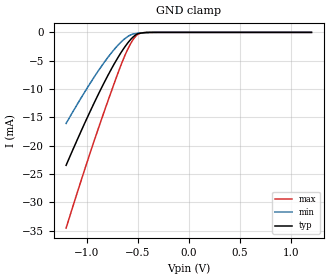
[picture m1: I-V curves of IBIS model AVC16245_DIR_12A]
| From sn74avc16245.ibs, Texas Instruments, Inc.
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[Model]   AVC16245_DIR_12A
Model_type  Input
Vinl = 0
Vinh = 1.2
| variable   typ   min   max
C_comp   1.77pF   1.45pF   1.99pF
[Temperature Range]   40   100   -40
| Ambient temperature   25   85   -40
[Voltage range]   1.2   1.2   1.2
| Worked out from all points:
|   GND clamp passes 1 mA (typ) near -0.56 V on its own axis
[GND Clamp]
| AVC16245_DIR_12A
|   Voltage   I(typ)   I(min)   I(max)
-1.2V     -23.48mA   -16.09mA   -34.58mA
-1.055V   -17.52mA   -11.63mA   -26.28mA
-920mV    -12.26mA   -7.746mA   -18.87mA
-800mV    -7.914mA   -4.632mA   -12.58mA
-700mV    -4.663mA   -2.414mA   -7.551mA
-640mV    -2.948mA   -1.337mA   -4.735mA
-590mV    -1.713mA   -656.6uA   -2.719mA
-545mV    -820.2uA   -290.5uA   -1.288mA
-505mV    -294.5uA   -174.3uA   -438.8uA
-455mV    -91.21uA   -79.33uA   -93.44uA
-385mV    -13.73uA   -21.91uA   -7.311uA
1.2V      671.7pA    3.121nA    23.8pA
